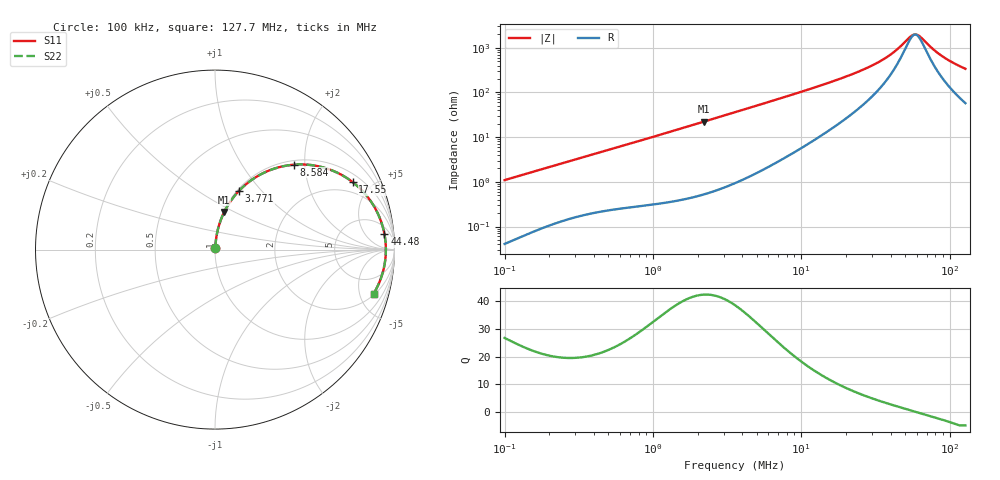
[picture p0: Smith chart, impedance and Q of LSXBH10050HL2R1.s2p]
! LSXBH10050HL2R1  S-PARAMETER MODEL  ( General Type )
! Model Generated by TAIYO YUDEN Corporation (http://www.ty-top.com)
! Version 3.0
! TAIYO YUDEN Control No. 180118NI43SB-FBB
! Copyright(c) 2007 TAIYO YUDEN CO.,LTD. All Rights Reserved.
! Product Description (link to TY-COMPAS)
! https://ds.yuden.co.jp/TYCOMPAS/or/detail?pn=LSXBH10050HL2R1N&u=M
! Products Name : Inductors
! Characteristics :
!  Inductance : 2.1 uH , SRF(min) : 37 MHz , DC Resistance(max) : 0.0104 Ohm
!  Rated Current : Saturation :10000 mA , Temp Rise : 8300 mA (40 degC)
!  Case Size : 10.0 x 9.8 / 0.394 x 0.386 [mm/inch] , Thickness : 5 / 0.197 [mm/inch]
!  (Conditions: Temperature = 25 degC , DC Bias Current/Voltage = 0A / 0V)
! External Node Assignments :
!  1  o---GGG---o  2
! GND o---------o GND
! Frequency Range : 0.1MHz  -  127.746476MHz  [ 402 STEP ]
# MHz S RI R 50
! Freq[MHz].  S11 Real  S11 Imag  S21 Real  S21 Imag  S12 Real  S12 Imag  S22 Real  S22 Imag
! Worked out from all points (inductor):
!   401 points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, 100 kHz to 127.7 MHz, reference 50 ohm
!   read as one part in series: L = 1.73 uH near 103.6 kHz
!   highest Q = 42.5 at 2.205 MHz (marker M1), where L = 1.61 uH
!   self-resonance near 58.64 MHz
!   S11 on the Smith chart (normalised r, x): 100 kHz: 1.00, +0.02; 3.771 MHz: 1.02, +0.76; 8.584 MHz: 1.08, +1.76; 17.55 MHz: 1.38, +3.84; 44.48 MHz: 10, +16; 127.7 MHz: 2.15, -6.67
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0.1  0.000528 0.0109  0.9995 -0.0109  0.9995 -0.0109  0.000528 0.0109
0.33137  0.00295 0.0345  0.9971 -0.0345  0.9971 -0.0345  0.00295 0.0345
1.098062  0.0153 0.1091  0.9847 -0.1091  0.9847 -0.1091  0.0153 0.1091
2.205443  0.0517 0.2099  0.9483 -0.2099  0.9483 -0.2099  0.0517 0.2099
3.574164  0.1216 0.3142  0.8784 -0.3142  0.8784 -0.3142  0.1216 0.3142
3.771135  0.1333 0.3269  0.8667 -0.3269  0.8667 -0.3269  0.1333 0.3269
5.588835  0.2507 0.417  0.7493 -0.417  0.7493 -0.417  0.2507 0.417
8.584247  0.4403 0.4731  0.5597 -0.4731  0.5597 -0.4731  0.4403 0.4731
11.84371  0.5996 0.4586  0.4004 -0.4586  0.4004 -0.4586  0.5996 0.4586
17.55242  0.7669 0.376  0.2331 -0.376  0.2331 -0.376  0.7669 0.376
27.9415  0.8908 0.2331  0.1092 -0.2331  0.1092 -0.2331  0.8908 0.2331
33.41246  0.9183 0.1756  0.0817 -0.1756  0.0817 -0.1756  0.9183 0.1756
39.24654  0.9354 0.1245  0.0646 -0.1245  0.0646 -0.1245  0.9354 0.1245
44.47976  0.9443 0.0853  0.0557 -0.0853  0.0557 -0.0853  0.9443 0.0853
55.12555  0.9516 0.019  0.0484 -0.019  0.0484 -0.019  0.9516 0.019
58.1635  0.952 0.00251  0.048 -0.00251  0.048 -0.00251  0.952 0.00251
60.28126  0.9519 -0.00848  0.0481 0.00848  0.0481 0.00848  0.9519 -0.00848
63.60334  0.9514 -0.025  0.0486 0.025  0.0486 0.025  0.9514 -0.025
76.0569  0.9452 -0.0802  0.0548 0.0802  0.0548 0.0802  0.9452 -0.0802
87.75374  0.9354 -0.125  0.0646 0.125  0.0646 0.125  0.9354 -0.125
106.8293  0.9135 -0.1876  0.0865 0.1876  0.0865 0.1876  0.9135 -0.1876
127.7465  0.884 -0.2452  0.116 0.2452  0.116 0.2452  0.884 -0.2452
